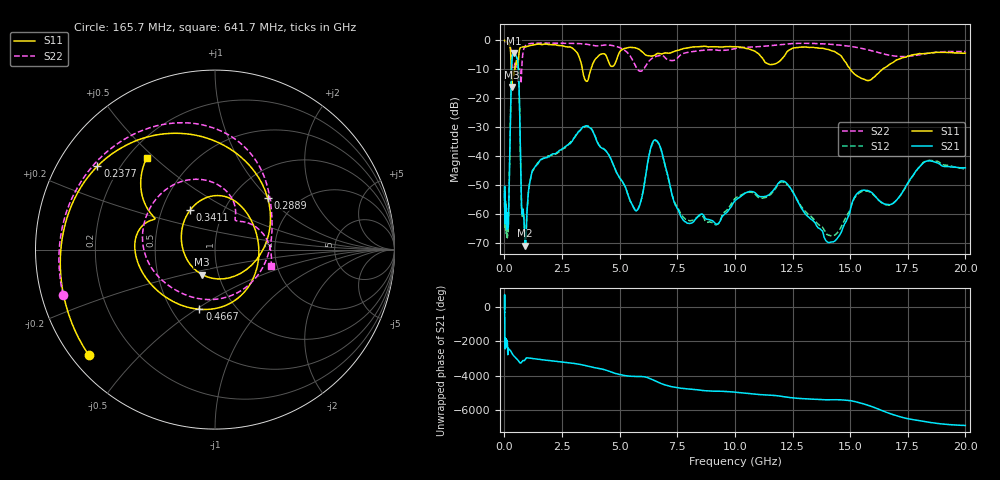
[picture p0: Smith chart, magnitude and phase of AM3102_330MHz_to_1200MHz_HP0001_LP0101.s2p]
! Date/Time: Tue, Sep 11, 2018 5:09 PM
! Network Analyzer: Agilent Technologies E8362B Rev: A.07.50.63
! Sweep from 0.010 to 20.000 GHz, 1601 Points, Sweep Type: LOG
! Power Supply: 4.950 V, 0.001 A
# Hz S DB R 50
!freq MagS11 AngS11 MagS21 AngS21 MagS12 AngS12 MagS22 AngS22
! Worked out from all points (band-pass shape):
!   1601 points, 10 MHz to 20 GHz, reference 50 ohm
!   highest |S21| = -4.29 dB at 414.5 MHz (marker M1); lowest = -70.9 dB at 907.7 MHz (marker M2)
!   |S21| within 3 dB of the highest: 321.9 MHz to 584.9 MHz (263 MHz wide, 58 % of centre)
!   lowest |S11| = -16.1 dB at 316.2 MHz (marker M3), VSWR 1.37, Z = 41.7 - j11.9 ohm
!   |S11| at or under -10 dB: 295.4 MHz to 451.1 MHz (155.7 MHz wide, 41.7 % of centre); 3.382 GHz to 3.755 GHz (373.1 MHz wide, 10.5 % of centre); 15.01 GHz to 16.4 GHz (1.393 GHz wide, 8.87 % of centre)
!   |S22| runs from -14.8 to -0.2 dB; largest |S21 - S12| = 0.01
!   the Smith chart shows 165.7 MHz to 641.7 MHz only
!   S11 on the Smith chart (normalised r, x): 165.7 MHz: 0.05, -0.36; 237.7 MHz: 0.12, +0.31; 288.9 MHz: 1.42, +0.99; 341.1 MHz: 0.69, +0.33; 466.7 MHz: 0.68, -0.51; 641.7 MHz: 0.27, +0.47
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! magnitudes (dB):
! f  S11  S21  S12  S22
! 10 MHz  0.0  -55.1  -53.9  -0.2
! 35.55 MHz  0.0  -58.6  -62.7  -0.4
! 126.4 MHz  -0.4  -63.5  -67.7  -0.9
! 165.7 MHz  -0.8  -63.5  -65.6  -1.1
! 237.7 MHz  -1.9  -37.1  -37.3  -1.8
! 288.9 MHz  -7.7  -15.1  -15.2  -3.9
! 316.2 MHz  -16.1  -8.1  -8.1  -7.4
! 341.1 MHz  -11.7  -5.8  -5.9  -10.2
! 414.5 MHz  -12.2  -4.3  -4.3  -9.7
! 447.2 MHz  -10.2  -4.5  -4.5  -8.2
! 466.7 MHz  -9.3  -4.7  -4.7  -7.7
! 641.7 MHz  -3.9  -17.4  -17.5  -9.8
! 750.6 MHz  -2.2  -58.2  -58.9  -10.4
! 907.7 MHz  -2.3  -70.9  -71.0  -1.9
! 1.59 GHz  -1.4  -41.1  -41.2  -0.9
! 3.651 GHz  -13.1  -29.8  -29.5  -1.4
! 5.652 GHz  -2.5  -58.4  -58.5  -8.2
! 6.549 GHz  -5.0  -34.4  -34.6  -5.6
! 7.882 GHz  -2.7  -62.8  -61.8  -4.2
! 12.09 GHz  -5.9  -48.6  -48.9  -1.3
! 14.14 GHz  -3.4  -69.7  -67.4  -1.3
! 20 GHz  -4.4  -44.0  -44.4  -3.8
